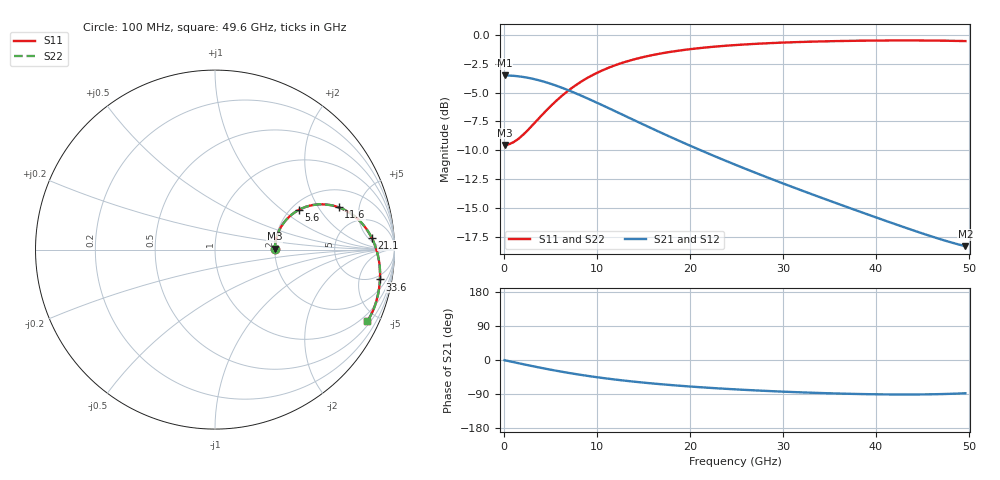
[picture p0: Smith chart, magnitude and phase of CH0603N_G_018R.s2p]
# GHz S RI R 18
! S-Parameters data
! Freq  reS11  imS11  reS21  imS21  reS12  imS12  reS22  imS22
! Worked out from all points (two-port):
!   100 points, 100 MHz to 49.6 GHz, reference 18 ohm
!   highest |S21| = -3.52 dB at 100 MHz (marker M1); lowest = -18.3 dB at 49.6 GHz (marker M2)
!   |S21| within 3 dB of the highest: start of sweep to 11.73 GHz
!   lowest |S11| = -9.5 dB at 100 MHz (marker M3), VSWR 2.00, Z = 36 + j0.41 ohm
!   |S11| at or under -10 dB: nowhere
!   |S22| runs from -9.5 to -0.5 dB; largest |S21 - S12| = 0
!   S11 on the Smith chart (normalised r, x): 100 MHz: 2.00, +0.02; 5.6 GHz: 2.20, +1.32; 11.6 GHz: 3.09, +3.10; 21.1 GHz: 11, +6; 33.6 GHz: 4, -10; 49.6 GHz: 0.66, -4.39
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0.1  0.3334 0.00506  0.6666 -0.00619  0.6666 -0.00619  0.3334 0.00506
1.1  0.3395 0.0551  0.6604 -0.0676  0.6604 -0.0676  0.3395 0.0551
1.6  0.3463 0.0793  0.6535 -0.0974  0.6535 -0.0974  0.3463 0.0793
2.6  0.3667 0.1244  0.6329 -0.1538  0.6329 -0.1538  0.3667 0.1244
4.1  0.411 0.1808  0.5879 -0.2271  0.5879 -0.2271  0.411 0.1808
5.6  0.4661 0.2208  0.5319 -0.2841  0.5319 -0.2841  0.4661 0.2208
7.1  0.5256 0.244  0.4711 -0.3242  0.4711 -0.3242  0.5256 0.244
8.6  0.5846 0.2523  0.4107 -0.3494  0.4107 -0.3494  0.5846 0.2523
10.1  0.6396 0.2484  0.3539 -0.3623  0.3539 -0.3623  0.6396 0.2484
11.6  0.6891 0.2354  0.3023 -0.366  0.3023 -0.366  0.6891 0.2354
14.1  0.7579 0.2  0.2294 -0.3585  0.2294 -0.3585  0.7579 0.2
16.6  0.8105 0.1552  0.172 -0.3413  0.172 -0.3413  0.8105 0.1552
18.6  0.8427 0.1162  0.1354 -0.3243  0.1354 -0.3243  0.8427 0.1162
21.1  0.8727 0.0663  0.0992 -0.3016  0.0992 -0.3016  0.8727 0.0663
25.1  0.9028 -0.0124  0.0577 -0.2659  0.0577 -0.2659  0.9028 -0.0124
29.1  0.9168 -0.0873  0.0304 -0.2332  0.0304 -0.2332  0.9168 -0.0873
33.1  0.9194 -0.1575  0.013 -0.2042  0.013 -0.2042  0.9194 -0.1575
33.6  0.919 -0.166  0.0113 -0.2008  0.0113 -0.2008  0.919 -0.166
37.6  0.9118 -0.2311  0.00168 -0.1758  0.00168 -0.1758  0.9118 -0.2311
41.6  0.8975 -0.2917  -0.00242 -0.1541  -0.00242 -0.1541  0.8975 -0.2917
46.6  0.8705 -0.3609  -0.000385 -0.1319  -0.000385 -0.1319  0.8705 -0.3609
49.6  0.8493 -0.3981  0.00487 -0.1219  0.00487 -0.1219  0.8493 -0.3981
